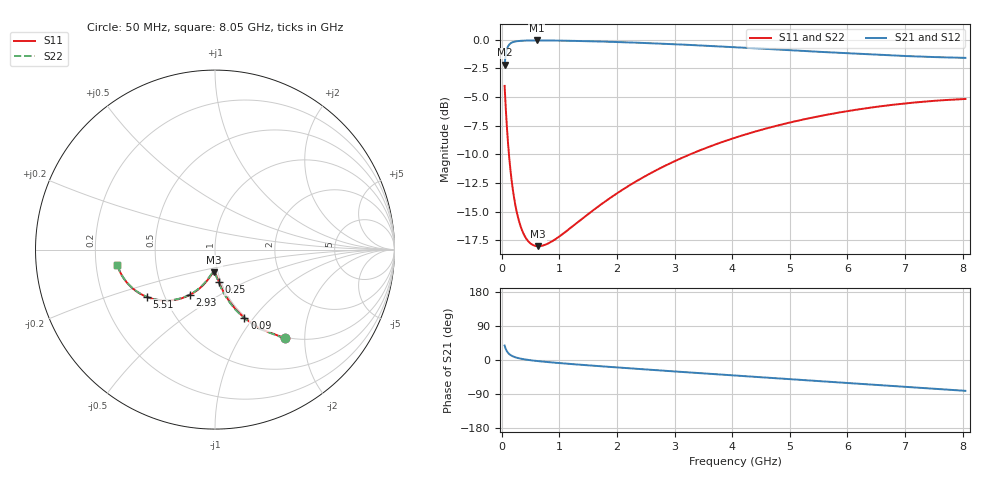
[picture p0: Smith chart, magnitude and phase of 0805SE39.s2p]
! AVX Thin Film Operation		Date: August 2001
! Description: Accu-P® Series, Thin Film, SMD, RF Capacitor
! Part Number: 08053K390FBT
! 50 MHz  -  8.05 GHz
! Serial Measurements
# mhz S db R 50
!	S11		S21		S12		S22
!	dB	Phase	dB	Phase	dB	Phase	dB	Phase
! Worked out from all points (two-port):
!   401 points, 50 MHz to 8.05 GHz, reference 50 ohm
!   highest |S21| = -0.07 dB at 610 MHz (marker M1); lowest = -2.2 dB at 50 MHz (marker M2)
!   |S21| within 3 dB of the highest: start of sweep to end of sweep
!   lowest |S11| = -18.0 dB at 630 MHz (marker M3), VSWR 1.29, Z = 48 - j12.2 ohm
!   |S11| at or under -10 dB: 125.4 MHz to 3.275 GHz (3.149 GHz wide, 185 % of centre)
!   |S22| runs from -18.0 to -4.0 dB; largest |S21 - S12| = 0
!   S11 on the Smith chart (normalised r, x): 50 MHz: 0.98, -1.60; 90 MHz: 0.98, -0.90; 250 MHz: 0.98, -0.37; 2.93 GHz: 0.67, -0.37; 5.51 GHz: 0.40, -0.27; 8.05 GHz: 0.29, -0.07
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50  -4.04 -51.8  -2.18 38.1  -2.18 38.1  -4.04 -51.9
90  -7.65 -66.8  -0.82 23.1  -0.82 23.1  -7.65 -67.1
110  -9.07 -71.0  -0.58 18.8  -0.58 18.8  -9.07 -71.3
130  -10.27 -74.0  -0.43 15.8  -0.43 15.8  -10.27 -74.4
150  -11.31 -76.3  -0.34 13.4  -0.34 13.4  -11.31 -76.8
190  -12.98 -79.7  -0.23 9.9  -0.23 9.9  -12.98 -80.3
250  -14.78 -83.1  -0.15 6.5  -0.15 6.5  -14.78 -83.8
330  -16.32 -86.0  -0.10 3.5  -0.10 3.5  -16.32 -86.8
410  -17.23 -88.1  -0.09 1.3  -0.09 1.3  -17.23 -89.0
510  -17.82 -90.2  -0.07 -0.8  -0.07 -0.8  -17.82 -91.2
610  -18.02 -92.0  -0.07 -2.6  -0.07 -2.6  -18.02 -93.0
630  -18.02 -92.3  -0.07 -2.9  -0.07 -2.9  -18.02 -93.3
890  -17.55 -96.1  -0.08 -6.7  -0.08 -6.7  -17.55 -97.0
1390  -15.65 -102.3  -0.12 -12.8  -0.12 -12.8  -15.65 -103.0
2070  -13.18 -109.9  -0.22 -20.3  -0.22 -20.3  -13.18 -110.5
2730  -11.27 -117.0  -0.34 -27.4  -0.34 -27.4  -11.27 -117.5
2930  -10.78 -119.1  -0.39 -29.5  -0.39 -29.5  -10.78 -119.5
4050  -8.56 -130.7  -0.66 -40.9  -0.66 -40.9  -8.56 -131.0
5390  -6.80 -144.2  -1.03 -54.4  -1.03 -54.4  -6.80 -144.4
5510  -6.68 -145.4  -1.06 -55.6  -1.06 -55.6  -6.68 -145.5
6730  -5.72 -157.6  -1.37 -67.8  -1.37 -67.8  -5.72 -157.7
8050  -5.18 -171.2  -1.59 -81.4  -1.59 -81.4  -5.18 -171.2
